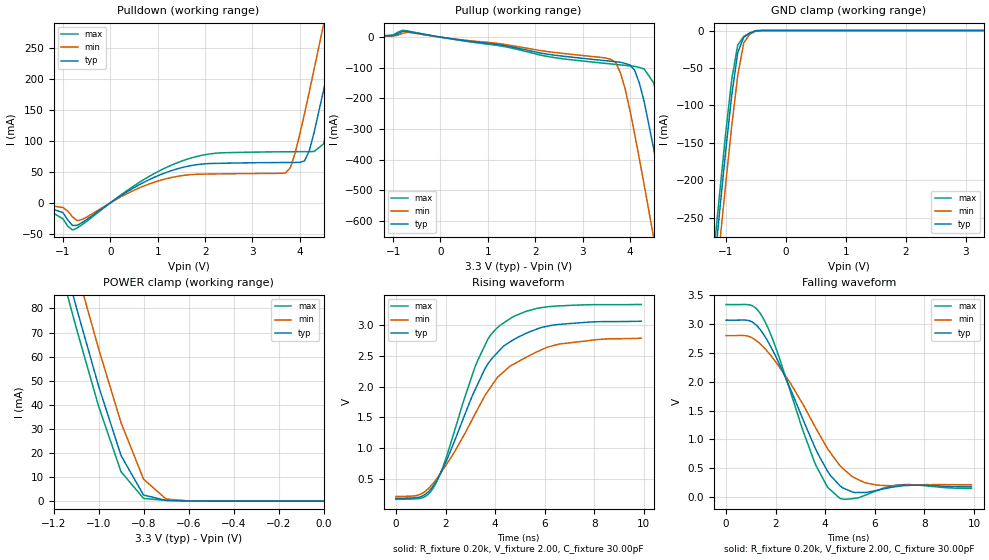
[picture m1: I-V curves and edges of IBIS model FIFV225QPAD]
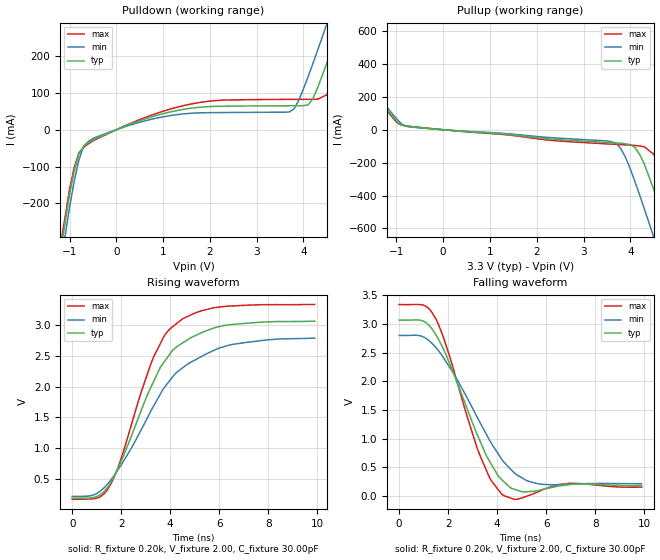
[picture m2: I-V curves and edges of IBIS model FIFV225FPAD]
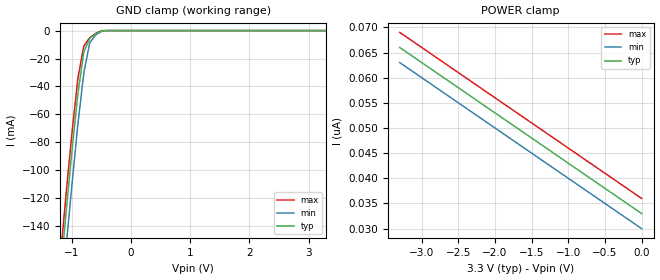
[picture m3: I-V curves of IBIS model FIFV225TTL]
| IBIS file i72v205.ibs created by s2ibis2 version 1.1
| North Carolina State University Electronics Research Laboratory  1995
[IBIS ver]   2.1
[File name]   i72v205.ibs
[File Rev]   1.0
[Date]   06/05/98
[Source]   Integrated Device Technology, Inc.
[Notes]   1. Temperatures: typ=25C, min=70C, max=0C 2. Cemos8_3.3V
   process. 3. Ramp rates based on 50 ohm load.
[Copyright]   Copyright 1998, Integrated Device Technology, Inc.
|   Component idt72V205
[Component]   idt72V205
[Manufacturer]   Integrated Device Technology
[Package]
| variable   typ   min   max
R_pkg   0.75   0.60   0.90
L_pkg   8.10nH   8.30nH   9.90nH
C_pkg   0.53pF   0.46pF   0.60pF
[Pin]  signal_name   model_name   R_pin   L_pin   C_pin
1   D15   FIFV225TTL
2   D14   FIFV225TTL
3   D13   FIFV225TTL
4   D12   FIFV225TTL
5   D11   FIFV225TTL
6   D10   FIFV225TTL
7   D9   FIFV225TTL
8   D8   FIFV225TTL
9   D7   FIFV225TTL
10   D6   FIFV225TTL
11   D5   FIFV225TTL
12   D4   FIFV225TTL
13   D3   FIFV225TTL
14   D2   FIFV225TTL
15   D1   FIFV225TTL
16   D0   FIFV225TTL
17   PAEL   FIFV225FPAD
18   FLB   FIFV225TTL
19   WCLK   FIFV225TTL
20   WENL   FIFV225TTL
21   WXIL   FIFV225TTL
22   VCC   POWER
23   PAFL   FIFV225FPAD
24   RXIL   FIFV225TTL
25   FFL   FIFV225FPAD
26   WXOLHF   FIFV225FPAD
27   RXOL   FIFV225FPAD
28   Q0   FIFV225QPAD
29   Q1   FIFV225QPAD
30   GND   GND
31   Q2   FIFV225QPAD
32   Q3   FIFV225QPAD
33   VCC   POWER
34   Q4   FIFV225QPAD
35   GND   GND
36   Q5   FIFV225QPAD
37   Q6   FIFV225QPAD
38   Q7   FIFV225QPAD
39   Q8   FIFV225QPAD
40   GND   GND
41   Q9   FIFV225QPAD
42   Q10   FIFV225QPAD
43   VCC   POWER
44   Q11   FIFV225QPAD
45   Q12   FIFV225QPAD
46   GND   GND
47   Q13   FIFV225QPAD
48   Q14   FIFV225QPAD
49   VCC   POWER
50   Q15   FIFV225QPAD
51   GND   GND
52   Q16   FIFV225QPAD
53   Q17   FIFV225QPAD
54   EFL   FIFV225FPAD
55   GND   GND
56   VCC   POWER
57   RSL   FIFV225TTL
58   OEL   FIFV225TTL
59   LDL   FIFV225TTL
60   RENL   FIFV225TTL
61   RCLK   FIFV225TTL
62   GND   GND
63   D17   FIFV225TTL
64   D16   FIFV225TTL
| Models and submodels in the file (3): FIFV225QPAD (3-state), FIFV225FPAD (Output), FIFV225TTL (Input)
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| FIN  FIN   dummy_model
| QIN  QIN   dummy_model
| QOEL QOEL   dummy_model
|   Model FIFV225QPAD
[Model]   FIFV225QPAD
Model_type   3-state
Polarity   Non-Inverting
Enable   Active-Low
Vmeas =  1.500V
C_comp   3.00pF   NA   NA
[Temperature Range]   25.00   70.00   0.000
[Voltage Range]   3.30V   3.00V   3.60V
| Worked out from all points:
|   slope of the pulldown table from 0 to 0.495 V, typ, clamps not added: 20.4 ohm
|   slope of the pullup table from 0 to 0.495 V, typ, clamps not added: 44.7 ohm
|   GND clamp passes 1 mA (typ) near -0.52 V on its own axis
|   POWER clamp passes 1 mA (typ) near -0.73 V on its own axis
|   rising waveform, R_fixture 0.20k, V_fixture 2.00, C_fixture 30.00pF: 20-80 % time 1.95ns typ, 2.41ns min, 1.64ns max; typ from 0.181 V to 3.07 V
|   falling waveform, R_fixture 0.20k, V_fixture 2.00, C_fixture 30.00pF: 20-80 % time 1.76ns typ, 2.17ns min, 1.5ns max; typ from 3.07 V to 0.177 V
[Pulldown]
| voltage   I(typ)   I(min)   I(max)
-3.3V     -1mA       -1mA       0A
-1.5V     -2.7mA     -2.1mA     -3.3mA
-800mV    -36.55mA   -22.69mA   -43.77mA
1.5V      56.64mA    43.75mA    67.16mA
3.7V      65mA       48.37mA    82.35mA
3.9V      65.11mA    80.12mA    82.43mA
4.1V      67.6mA     144mA      82.48mA
4.5V      181mA      287mA      94.75mA
4.7V      253mA      361mA      155mA
4.9V      326mA      435mA      225mA
5.1V      400mA      510mA      298mA
6.6V      966mA      1.076A     862mA
[Pullup]
| voltage   I(typ)   I(min)   I(max)
-3.3V     300uA      300uA      300uA
-800mV    19.13mA    12.44mA    22.38mA
3.6V      -78.68mA   -72.88mA   -87.52mA
3.7V      -80.24mA   -82.94mA   -89.09mA
3.9V      -85.87mA   -170mA     -92.22mA
4.1V      -108mA     -317mA     -95.4mA
4.3V      -210mA     -482mA     -104mA
4.5V      -363mA     -653mA     -149mA
4.7V      -531mA     -826mA     -270mA
4.9V      -703mA     -1A        -430mA
5.1V      -878mA     -1.176A    -601mA
6.6V      -2.207A    -2.508A    -1.926A
[GND_clamp]
| voltage   I(typ)   I(min)   I(max)
-3.3V     -2.171A    -2.212A    -2.149A
-1.2V     -323mA     -367mA     -298mA
-1.1V     -240mA     -284mA     -216mA
-1V       -160mA     -204mA     -136mA
-900mV    -86.07mA   -127mA     -65.05mA
-800mV    -29.34mA   -59.59mA   -19.24mA
-700mV    -8.788mA   -16.49mA   -7.804mA
-600mV    -3.672mA   -4.887mA   -3.17mA
-500mV    -365uA     -944uA     -138uA
-400mV    -14.29nA   -611nA     -4.611nA
3.3V      33nA       33.88nA    33nA
[POWER_clamp]
| voltage   I(typ)   I(min)   I(max)
-3.3V     901mA      915mA      893mA
-1.2V     116mA      132mA      107mA
-1.1V     80.92mA    96.84mA    72.29mA
-1V       47.89mA    63.39mA    39.51mA
-900mV    18.95mA    32.6mA     12.21mA
-800mV    2.533mA    9.147mA    1.14mA
-700mV    314uA      878uA      268uA
-600mV    64.82uA    96.03uA    58.5uA
0V        33nA       30nA       36nA
[Ramp]
| variable   typ   min   max
dV/dt_r   1.03/1.09n   0.87/1.27n   1.19/0.99n
dV/dt_f   1.35/1.45n   1.13/1.85n   1.54/1.17n
R_load = 50.00
[Rising Waveform]
R_fixture = 0.20k
V_fixture = 2.00
C_fixture = 30.00pF
R_dut = 0.75
L_dut = 8.10nH
C_dut = 0.53pF
| time   V(typ)   V(min)   V(max)
0s        181mV      211mV      165mV
1ns       207mV      250mV      183mV
1.5ns     380mV      424mV      346mV
2ns       761mV      708mV      812mV
3.2ns     1.956V     1.561V     2.333V
3.7ns     2.364V     1.92V      2.767V
4.2ns     2.601V     2.19V      2.998V
5.2ns     2.859V     2.468V     3.22V
6.4ns     3.007V     2.675V     3.312V
9.9ns     3.067V     2.791V     3.339V
[Falling Waveform]
R_fixture = 0.20k
V_fixture = 2.00
C_fixture = 30.00pF
R_dut = 0.75
L_dut = 8.10nH
C_dut = 0.53pF
| time   V(typ)   V(min)   V(max)
0s        3.068V     2.8V       3.338V
1ns       3.048V     2.773V     3.327V
1.5ns     2.831V     2.606V     3.1V
2ns       2.445V     2.345V     2.598V
3.6ns     846mV      1.212V     571mV
4.1ns     445mV      835mV      168mV
4.6ns     195mV      542mV      -23.03mV
6.1ns     119mV      207mV      115mV
7.3ns     201mV      207mV      218mV
9.9ns     177mV      213mV      152mV
|   Model FIFV225FPAD
[Model]   FIFV225FPAD
Model_type   Output
Vmeas =  1.500V
C_comp   3.00pF   NA   NA
[Temperature Range]   25.00   70.00   0.000
[Voltage Range]   3.30V   3.00V   3.60V
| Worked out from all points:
|   slope of the pulldown table from 0 to 0.495 V, typ, clamps not added: 20.4 ohm
|   slope of the pullup table from 0 to 0.495 V, typ, clamps not added: 44.7 ohm
|   rising waveform, R_fixture 0.20k, V_fixture 2.00, C_fixture 30.00pF: 20-80 % time 1.94ns typ, 2.4ns min, 1.63ns max; typ from 0.181 V to 3.07 V
|   falling waveform, R_fixture 0.20k, V_fixture 2.00, C_fixture 30.00pF: 20-80 % time 1.62ns typ, 2.05ns min, 1.36ns max; typ from 3.07 V to 0.176 V
[Pulldown]
| voltage   I(typ)   I(min)   I(max)
-3.3V     -2.793A    -2.213A    -2.149A
-1.5V     -582mA     -626mA     -558mA
-1V       -176mA     -211mA     -162mA
-800mV    -65.89mA   -82.28mA   -63.01mA
-400mV    -21.63mA   -18.48mA   -23.86mA
1.6V      58.46mA    44.74mA    69.8mA
3.7V      65mA       48.37mA    82.35mA
4.1V      67.6mA     144mA      82.48mA
4.5V      181mA      287mA      94.75mA
4.7V      253mA      361mA      155mA
5.1V      400mA      510mA      298mA
6.6V      966mA      1.076A     862mA
[Pullup]
| voltage   I(typ)   I(min)   I(max)
-3.3V     901mA      915mA      893mA
-2.5V     598mA      613mA      590mA
-900mV    29.8mA     38.77mA    28.31mA
3.6V      -78.68mA   -72.88mA   -87.52mA
3.9V      -85.87mA   -170mA     -92.22mA
4.1V      -108mA     -317mA     -95.4mA
4.3V      -210mA     -482mA     -104mA
4.5V      -363mA     -653mA     -149mA
4.7V      -531mA     -826mA     -270mA
4.9V      -703mA     -1A        -430mA
5.1V      -878mA     -1.176A    -601mA
6.6V      -2.207A    -2.508A    -1.926A
[Ramp]
| variable   typ   min   max
dV/dt_r   1.03/1.07n   0.87/1.29n   1.19/0.96n
dV/dt_f   1.35/1.23n   1.13/1.60n   1.54/1.03n
R_load = 50.00
[Rising Waveform]
R_fixture = 0.20k
V_fixture = 2.00
C_fixture = 30.00pF
R_dut = 0.75
L_dut = 8.10nH
C_dut = 0.53pF
| time   V(typ)   V(min)   V(max)
0s        181mV      211mV      165mV
1ns       210mV      260mV      183mV
1.5ns     393mV      443mV      363mV
2ns       788mV      728mV      837mV
3.3ns     2.067V     1.67V      2.468V
3.8ns     2.43V      2.009V     2.856V
4.1ns     2.595V     2.161V     2.978V
5.1ns     2.846V     2.454V     3.213V
6.4ns     3.009V     2.676V     3.312V
9.9ns     3.067V     2.791V     3.339V
[Falling Waveform]
R_fixture = 0.20k
V_fixture = 2.00
C_fixture = 30.00pF
R_dut = 0.75
L_dut = 8.10nH
C_dut = 0.53pF
| time   V(typ)   V(min)   V(max)
0s        3.068V     2.8V       3.338V
1ns       3.047V     2.771V     3.327V
1.5ns     2.812V     2.59V      3.088V
3.2ns     1.059V     1.362V     814mV
3.7ns     598mV      964mV      309mV
4.2ns     280mV      631mV      25.41mV
5ns       74.15mV    319mV      -37.61mV
5.7ns     96.8mV     209mV      77.59mV
7ns       200mV      204mV      221mV
9.9ns     176mV      212mV      154mV
|   Model FIFV225TTL
[Model]   FIFV225TTL
Model_type   Input
Vinl =  0.000V
Vinh =  3.000V
Vmeas =  1.500V
C_comp   3.00pF   NA   NA
[Temperature Range]   25.00   70.00   0.000
[Voltage Range]   3.30V   3.00V   3.60V
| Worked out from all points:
|   GND clamp passes 1 mA (typ) near -0.54 V on its own axis
[GND_clamp]
| voltage   I(typ)   I(min)   I(max)
-3.3V     -1.215A    -1.238A    -1.203A
-1.2V     -177mA     -201mA     -164mA
-1.1V     -130mA     -155mA     -117mA
-1V       -85.9mA    -110mA     -73.09mA
-900mV    -45.15mA   -67.03mA   -34.14mA
-800mV    -15.42mA   -30.38mA   -11.05mA
-700mV    -5.554mA   -8.773mA   -5.066mA
-600mV    -2.384mA   -3.102mA   -2.034mA
-500mV    -209uA     -595uA     -61.81uA
-400mV    -8.386nA   -263nA     -4.26nA
3.3V      33nA       33nA       33nA
[POWER_clamp]
| voltage   I(typ)   I(min)   I(max)
-3.3V     66nA       63nA       69nA
-3.2V     65nA       62nA       68nA
-3V       63nA       60nA       66nA
0V        33nA       30nA       36nA
